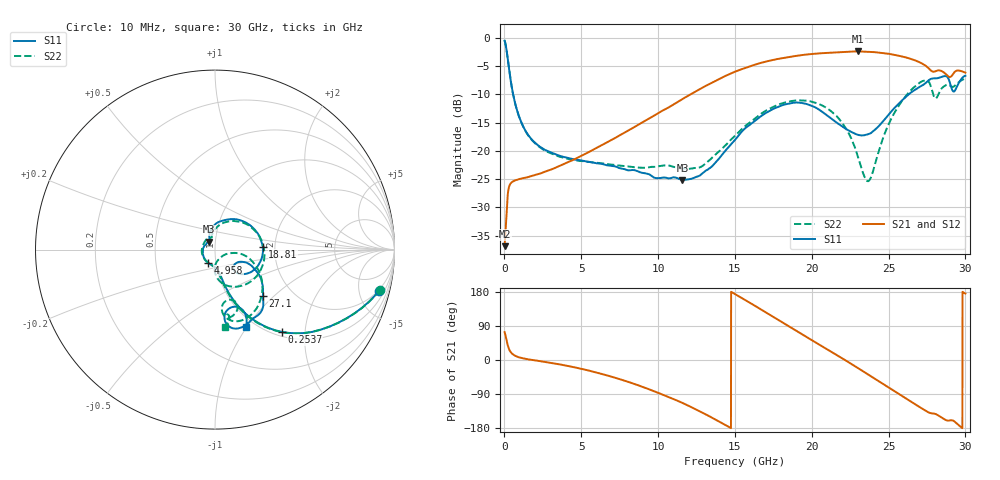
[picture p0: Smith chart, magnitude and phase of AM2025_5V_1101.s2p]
!Keysight Technologies,N5245B,MY58422270,A.16.20.02
!Date: Tuesday, July 14, 2026 01:10:27
!Correction: S11(C  2-Port  )
!S21(C  2-Port  )
!S12(C  2-Port  )
!S22(C  2-Port  )
!S2P File: Measurements: S11, S21, S12, S22:
# Hz S  dB  R 50
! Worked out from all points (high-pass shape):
!   3201 points, 10 MHz to 30 GHz, reference 50 ohm
!   highest |S21| = -2.42 dB at 23.03 GHz (marker M1); lowest = -36.9 dB at 10 MHz (marker M2)
!   |S21| within 3 dB of the highest: 15.6 GHz to 27.61 GHz (12.01 GHz wide, 55.6 % of centre)
!   lowest |S11| = -25.1 dB at 11.58 GHz (marker M3), VSWR 1.12, Z = 46.6 + j4.16 ohm
!   |S11| at or under -10 dB: 564.1 MHz to 26.32 GHz (25.76 GHz wide, 192 % of centre)
!   |S22| runs from -25.4 to -0.5 dB; largest |S21 - S12| = 0.0031
!   S11 on the Smith chart (normalised r, x): 10 MHz: 1.87, -7.64; 253.7 MHz: 1.08, -1.52; 4.958 GHz: 0.92, -0.13; 18.81 GHz: 1.72, +0.06; 27.1 GHz: 1.42, -0.86; 30 GHz: 0.90, -0.99
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1e7  -0.52 -14.1  -36.85 73.5  -38.23 63.4  -0.48 -13.9
2.536688e8  -4.57 -50.9  -26.90 33.5  -26.90 33.4  -4.60 -51.2
6.098e8  -10.59 -70.1  -25.33 13.3  -25.26 12.9  -10.61 -70.8
1.612591e9  -17.46 -79.2  -24.58 1.3  -24.57 1.3  -17.53 -80.8
4.95835e9  -21.66 -118.3  -20.95 -22.8  -20.92 -22.8  -21.79 -124.3
5.014581e9  -21.69 -119.3  -20.87 -23.4  -20.84 -23.3  -21.80 -125.4
1.000979e10  -24.83 150.9  -13.33 -86.6  -13.33 -86.6  -22.74 138.2
1.158427e10  -25.14 126.5  -10.85 -113.3  -10.84 -113.4  -23.12 110.8
1.336492e10  -23.05 116.6  -8.14 -149.1  -8.14 -149.2  -21.61 101.7
1.5005e10  -18.06 95.6  -6.00 174.0  -6.01 174.0  -17.35 81.2
1.67388e10  -13.79 55.8  -4.41 132.3  -4.41 132.2  -13.38 45.2
1.880998e10  -11.50 3.7  -3.28 81.6  -3.28 81.5  -11.14 -6.7
2.000958e10  -12.04 -24.6  -2.87 52.2  -2.87 52.2  -11.31 -36.4
2.16028e10  -14.97 -46.8  -2.58 13.6  -2.57 13.6  -13.82 -74.3
2.302732e10  -17.18 -41.7  -2.42 -21.8  -2.41 -21.8  -21.28 -89.1
2.373959e10  -16.99 -31.4  -2.47 -39.9  -2.47 -40.0  -25.24 -41.6
2.500479e10  -13.60 -23.0  -2.83 -72.5  -2.84 -72.6  -15.28 -11.5
2.710409e10  -8.56 -44.3  -4.46 -126.3  -4.45 -126.4  -7.83 -56.7
2.758206e10  -7.59 -50.1  -5.34 -137.9  -5.34 -138.1  -7.67 -74.9
2.806939e10  -7.18 -60.4  -5.91 -142.7  -5.90 -142.7  -10.74 -74.7
2.902532e10  -8.25 -82.1  -6.93 -159.2  -6.92 -159.4  -8.52 -79.9
3e10  -6.71 -68.2  -6.17 175.4  -6.16 175.3  -7.21 -82.9
